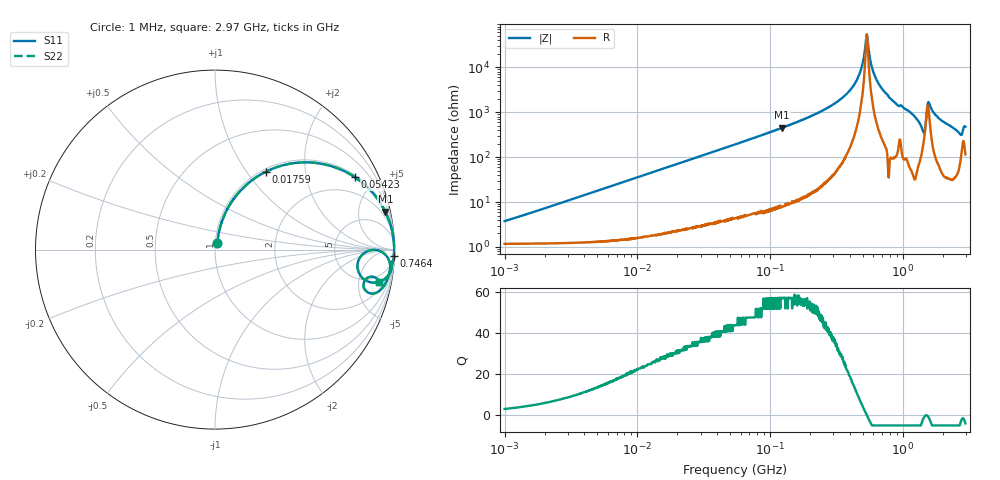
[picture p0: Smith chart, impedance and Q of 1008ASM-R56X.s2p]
!s-Parameter Generated by FASTRON Sdn. Bhd.
!FASTRON P/N : 1008ASM-R56X
!Keysight Technologies: E4991B_MY54100416_A.01.15
!Date: Tue Nov 21 09:20:58 2023
!Version  :Rev00  Wed Nov 22 15:16:01 2023
!Data & Calibration Information:
!Freq  S11  S21  S12  S22
!PortZ  Port1:50+j0  Port2:50+j0
!When reading reference impedance value at option line is always used.
! Remarks : This data is being provided solely for informational purposes.
# Hz S dB R 50
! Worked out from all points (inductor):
!   1599 points, 1 MHz to 2.97 GHz, reference 50 ohm
!   read as one part in series: L = 569 nH near 1.036 MHz
!   highest Q = 57.3 at 123.8 MHz (marker M1), where L = 578 nH
!   self-resonance near 536.5 MHz
!   S11 on the Smith chart (normalised r, x): 1 MHz: 1.02, +0.07; 17.59 MHz: 1.04, +1.24; 54.23 MHz: 1.09, +3.81; 746.4 MHz: 4, -53; 2.97 GHz: 3.28, -9.13
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1000000  -28.60 69.8  -0.11 -2.0  -0.11 -2.0  -28.60 69.8
3804036  -17.50 77.1  -0.18 -7.6  -0.18 -7.6  -17.50 77.1
1.439846e7  -6.99 61.3  -1.13 -26.5  -1.13 -26.5  -6.99 61.3
1.758912e7  -5.69 56.8  -1.55 -31.3  -1.55 -31.3  -5.69 56.8
5.422683e7  -1.14 27.4  -6.73 -61.3  -6.73 -61.3  -1.14 27.4
5.477226e7  -1.12 27.2  -6.80 -61.5  -6.80 -61.5  -1.12 27.2
1.238204e8  -0.24 12.5  -13.30 -76.5  -13.30 -76.5  -0.24 12.5
2.073156e8  -0.08 6.8  -18.50 -82.1  -18.50 -82.1  -0.08 6.8
3.172153e8  -0.03 3.4  -24.50 -84.9  -24.50 -84.9  -0.03 3.4
4.135554e8  -0.02 1.7  -30.80 -84.9  -30.80 -84.9  -0.02 1.7
4.805402e8  -0.02 0.7  -38.20 -80.9  -38.20 -80.9  -0.02 0.7
5.364635e8  -0.02 0.0  -54.60 -2.8  -54.60 -2.8  -0.02 0.0
6.110031e8  -0.02 -0.8  -36.70 81.2  -36.70 81.2  -0.02 -0.8
7.463997e8  -0.03 -2.2  -28.50 84.3  -28.50 84.3  -0.03 -2.2
7.846996e8  -0.02 -2.6  -26.90 86.5  -26.90 86.5  -0.02 -2.6
1.176881e9  -0.10 -6.2  -19.30 81.0  -19.30 81.0  -0.10 -6.2
1.416254e9  -1.02 -11.9  -13.00 54.7  -13.00 54.7  -1.02 -11.9
1.45942e9  -1.95 -7.0  -12.80 25.2  -12.80 25.2  -1.95 -7.0
1.581072e9  -0.31 -2.8  -24.40 52.9  -24.40 52.9  -0.31 -2.8
1.902655e9  -0.18 -8.0  -17.10 77.4  -17.10 77.4  -0.18 -8.0
2.660507e9  -0.70 -15.3  -11.50 65.6  -11.50 65.6  -0.70 -15.3
2.970126e9  -0.60 -11.1  -14.10 64.9  -14.10 64.9  -0.60 -11.1
